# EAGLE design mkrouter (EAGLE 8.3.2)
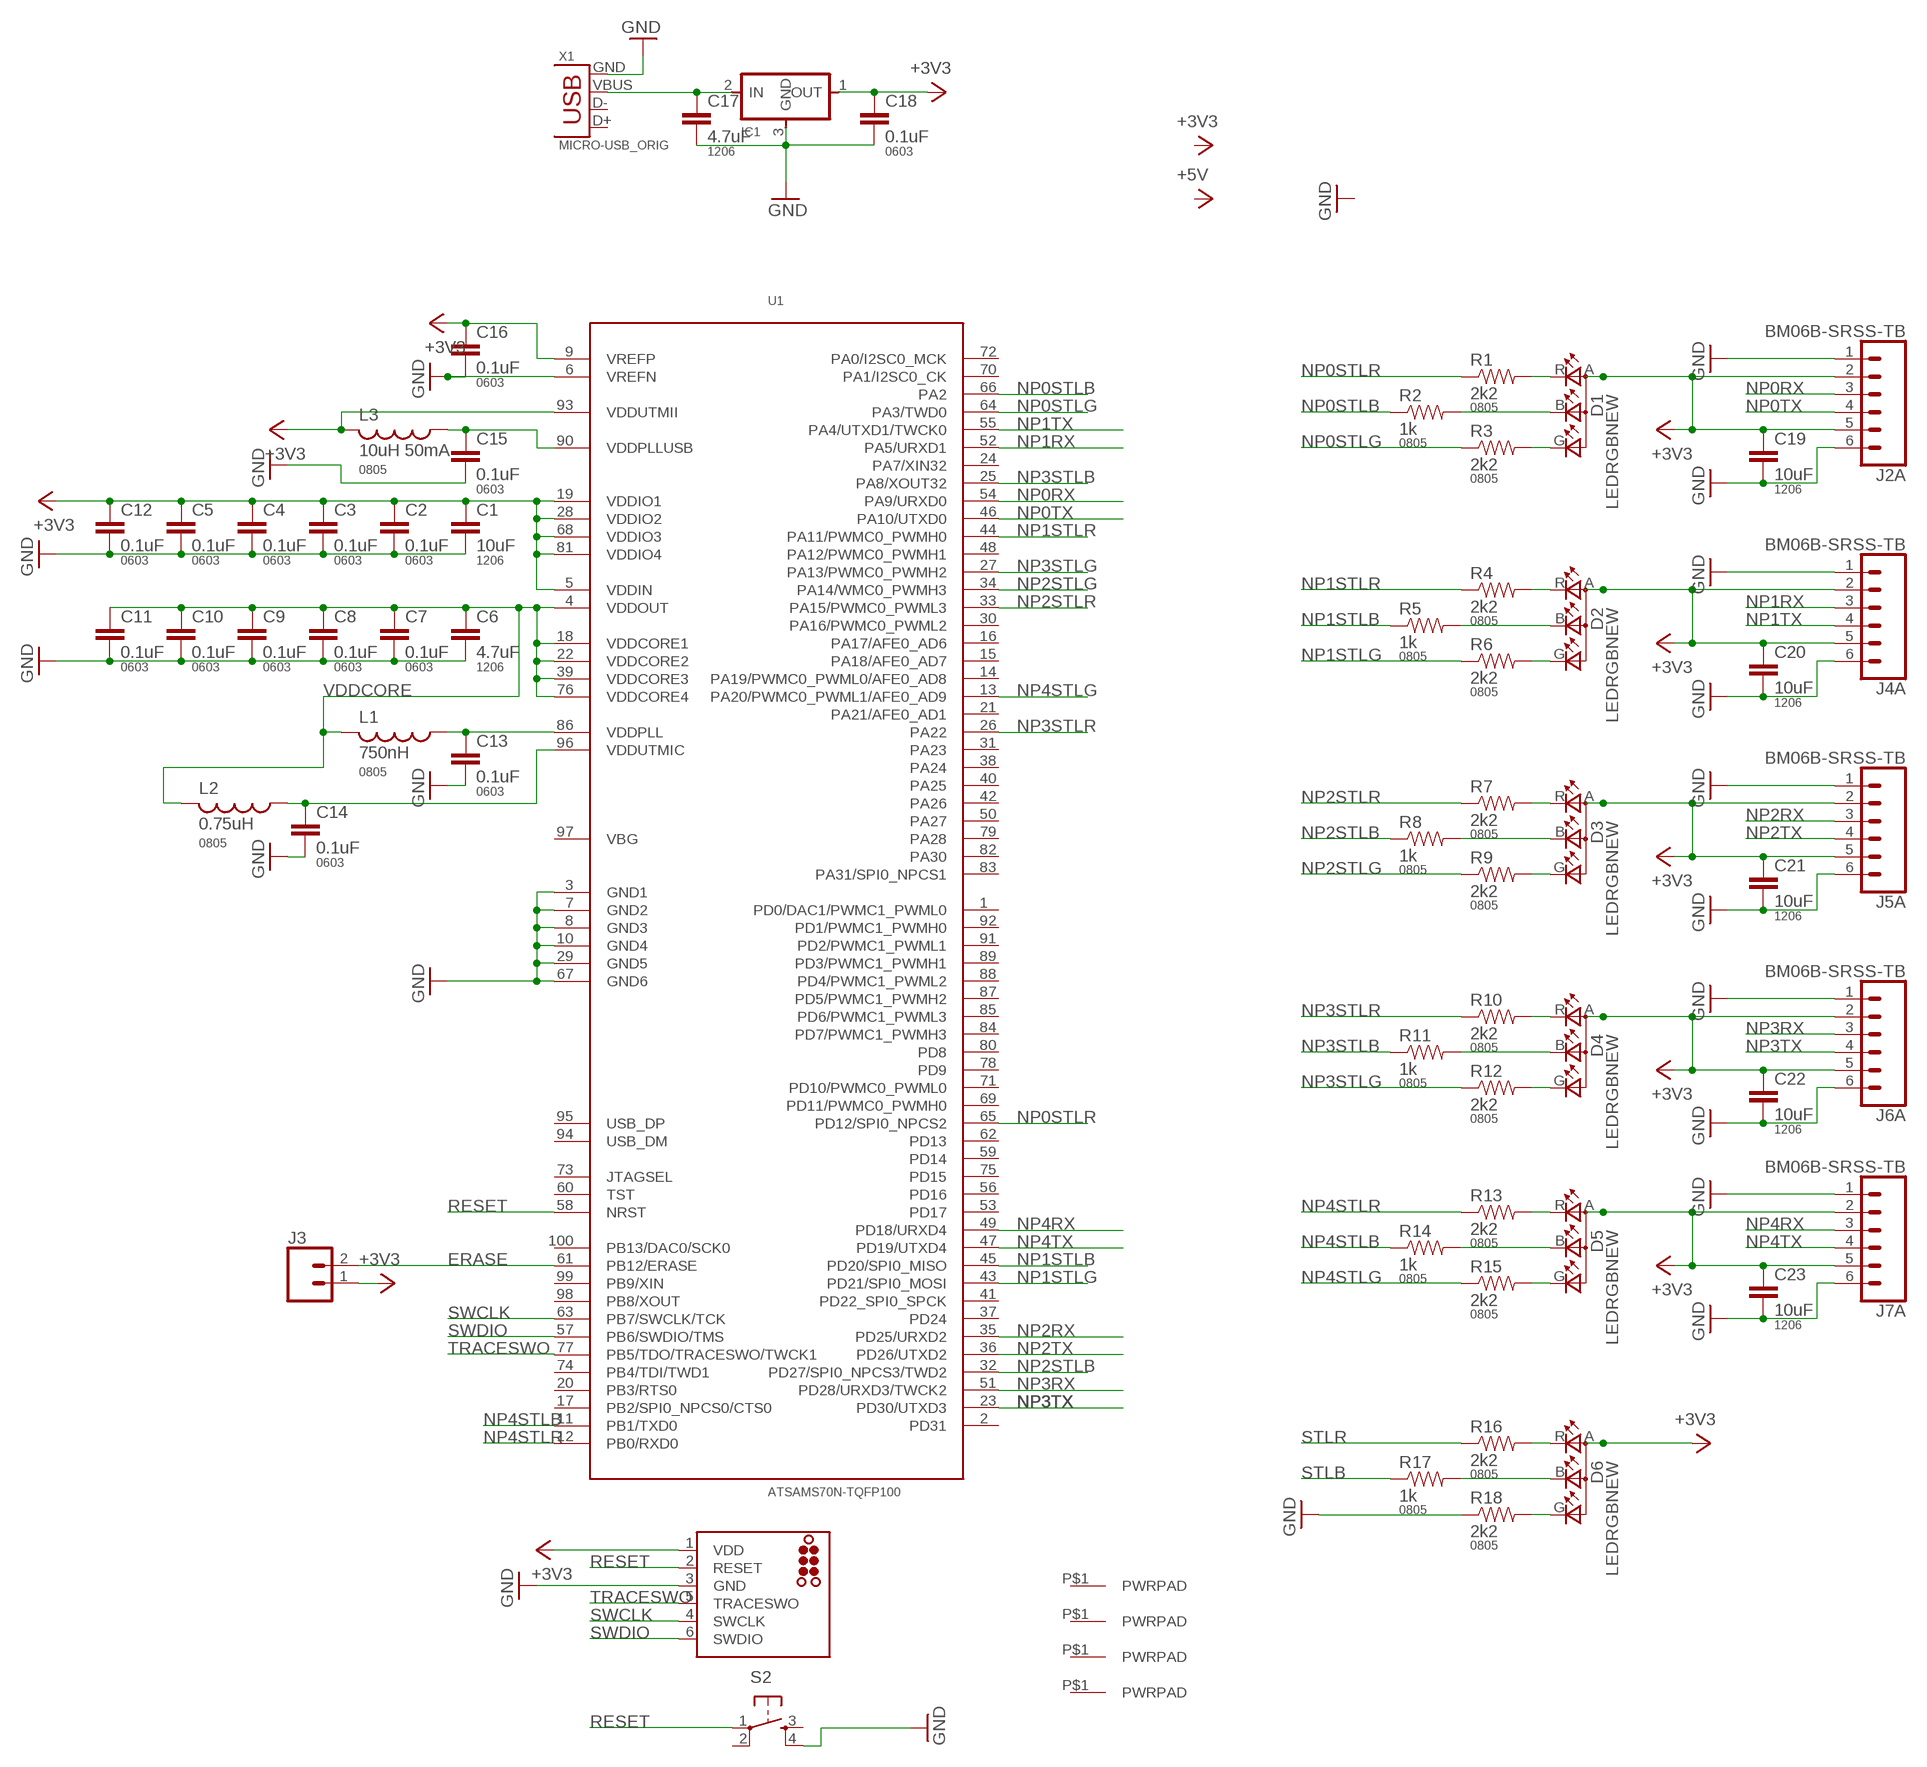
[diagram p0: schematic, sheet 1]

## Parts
C1  10uF  CAP1206  [1206]
C2  0.1uF  CAP0603-CAP  [0603-CAP]
C3  0.1uF  CAP0603-CAP  [0603-CAP]
C4  0.1uF  CAP0603-CAP  [0603-CAP]
C5  0.1uF  CAP0603-CAP  [0603-CAP]
C6  4.7uF  CAP1206  [1206]
C7  0.1uF  CAP0603-CAP  [0603-CAP]
C8  0.1uF  CAP0603-CAP  [0603-CAP]
C9  0.1uF  CAP0603-CAP  [0603-CAP]
C10  0.1uF  CAP0603-CAP  [0603-CAP]
C11  0.1uF  CAP0603-CAP  [0603-CAP]
C12  0.1uF  CAP0603-CAP  [0603-CAP]
C13  0.1uF  CAP0603-CAP  [0603-CAP]
C14  0.1uF  CAP0603-CAP  [0603-CAP]
C15  0.1uF  CAP0603-CAP  [0603-CAP]
C16  0.1uF  CAP0603-CAP  [0603-CAP]
C17  4.7uF  CAP1206  [1206]
C18  0.1uF  CAP0603-CAP  [0603-CAP]
C19  10uF  CAP1206  [1206]
C20  10uF  CAP1206  [1206]
C21  10uF  CAP1206  [1206]
C22  10uF  CAP1206  [1206]
C23  10uF  CAP1206  [1206]
D1  LEDRGBNEW  [P-LCC-4]
D2  LEDRGBNEW  [P-LCC-4]
D3  LEDRGBNEW  [P-LCC-4]
D4  LEDRGBNEW  [P-LCC-4]
D5  LEDRGBNEW  [P-LCC-4]
D6  LEDRGBNEW  [P-LCC-4]
IC1  REGULATORSOT23  [SOT23]
J1  TC2030-SWD-MCP  [TC2030-MCP]
J2  BM06B-SRSS-TB  JST_6_PIN_HORIZONTAL  [JST-6-SMD-HORI-1.0MM]
J3  CONN_021X02_NO_SILK  [1X02_NO_SILK]
J4  BM06B-SRSS-TB  JST_6_PIN_HORIZONTAL  [JST-6-SMD-HORI-1.0MM]
J5  BM06B-SRSS-TB  JST_6_PIN_HORIZONTAL  [JST-6-SMD-HORI-1.0MM]
J6  BM06B-SRSS-TB  JST_6_PIN_HORIZONTAL  [JST-6-SMD-HORI-1.0MM]
J7  BM06B-SRSS-TB  JST_6_PIN_HORIZONTAL  [JST-6-SMD-HORI-1.0MM]
J8  PWRPADM3  [PWRPAD_3-25MM]
J9  PWRPADM3  [PWRPAD_3-25MM]
J10  PWRPADM3  [PWRPAD_3-25MM]
J11  PWRPADM3  [PWRPAD_3-25MM]
L1  750nH  INDUCTOR-0805  [0805]
L2  0.75uH  INDUCTOR-0805  [0805]
L3  10uH 50mA  INDUCTOR-0805  [0805]
R1  2k2  RESISTOR0805-RES  [0805]
R2  1k  RESISTOR0805-RES  [0805]
R3  2k2  RESISTOR0805-RES  [0805]
R4  2k2  RESISTOR0805-RES  [0805]
R5  1k  RESISTOR0805-RES  [0805]
R6  2k2  RESISTOR0805-RES  [0805]
R7  2k2  RESISTOR0805-RES  [0805]
R8  1k  RESISTOR0805-RES  [0805]
R9  2k2  RESISTOR0805-RES  [0805]
R10  2k2  RESISTOR0805-RES  [0805]
R11  1k  RESISTOR0805-RES  [0805]
R12  2k2  RESISTOR0805-RES  [0805]
R13  2k2  RESISTOR0805-RES  [0805]
R14  1k  RESISTOR0805-RES  [0805]
R15  2k2  RESISTOR0805-RES  [0805]
R16  2k2  RESISTOR0805-RES  [0805]
R17  1k  RESISTOR0805-RES  [0805]
R18  2k2  RESISTOR0805-RES  [0805]
S2  6MM_SWITCH6MM_SWITCH  [6MM_SWITCH]
U1  ATSAMS70N-TQFP100  [TQFP100-14X14]
X1  MICRO-USB_ORIG  [DX4R005HJ5]

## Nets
+3V3: C1.1 C2.1 C3.1 C4.1 C5.1 C12.1 C16.1 C18.1 C19.1 C20.1 C21.1 C22.1 C23.1 D1.A(A2) D2.A(A2) D3.A(A2) D4.A(A2) D5.A(A2) D6.A(A2) IC1.1(OUT) J1.1(VDD) J2.2 J2.5 J3.1 J4.2 J4.5 J5.2 J5.5 J6.2 J6.5 J7.2 J7.5 L3.2 U1.5(VDDIN) U1.9(VREFP) U1.19(VDDIO1) U1.28(VDDIO2) U1.68(VDDIO3) U1.81(VDDIO4) U1.93(VDDUTMII)
ERASE: J3.2 U1.61(PB12/ERASE)
GND: C1.2 C2.2 C3.2 C4.2 C5.2 C6.2 C7.2 C8.2 C9.2 C10.2 C11.2 C12.2 C13.2 C14.2 C15.2 C16.2 C17.2 C18.2 C19.2 C20.2 C21.2 C22.2 C23.2 IC1.3(GND) J1.3(GND) J2.1 J2.6 J4.1 J4.6 J5.1 J5.6 J6.1 J6.6 J7.1 J7.6 R18.1 S2.4(S1) U1.3(GND1) U1.6(VREFN) U1.7(GND2) U1.8(GND3) U1.10(GND4) U1.29(GND5) U1.67(GND6) X1.GND
N$1: C13.1 L1.1 U1.86(VDDPLL)
N$2: D1.R(CRED) R1.2
N$3: C14.1 L2.1 U1.96(VDDUTMIC)
N$4: C17.1 IC1.2(IN) X1.VBUS
N$5: C15.1 L3.1 U1.90(VDDPLLUSB)
N$6: D1.B(CBLUE) R2.2
N$7: D1.G(CGREEN) R3.2
N$8: D2.R(CRED) R4.2
N$9: D2.B(CBLUE) R5.2
N$10: D2.G(CGREEN) R6.2
N$11: D3.R(CRED) R7.2
N$12: D3.B(CBLUE) R8.2
N$13: D3.G(CGREEN) R9.2
N$14: D4.R(CRED) R10.2
N$15: D4.B(CBLUE) R11.2
N$16: D4.G(CGREEN) R12.2
N$17: D5.R(CRED) R13.2
N$18: D5.B(CBLUE) R14.2
N$19: D5.G(CGREEN) R15.2
N$20: D6.R(CRED) R16.2
N$21: D6.B(CBLUE) R17.2
N$22: D6.G(CGREEN) R18.2
NP0RX: J2.3 U1.54(PA9/URXD0)
NP0STLB: R2.1 U1.66(PA2)
NP0STLG: R3.1 U1.64(PA3/TWD0)
NP0STLR: R1.1 U1.65(PD12/SPI0_NPCS2)
NP0TX: J2.4 U1.46(PA10/UTXD0)
NP1RX: J4.3 U1.52(PA5/URXD1)
NP1STLB: R5.1 U1.45(PD20/SPI0_MISO)
NP1STLG: R6.1 U1.43(PD21/SPI0_MOSI)
NP1STLR: R4.1 U1.44(PA11/PWMC0_PWMH0)
NP1TX: J4.4 U1.55(PA4/UTXD1/TWCK0)
NP2RX: J5.3 U1.35(PD25/URXD2)
NP2STLB: R8.1 U1.32(PD27/SPI0_NPCS3/TWD2)
NP2STLG: R9.1 U1.34(PA14/WMC0_PWMH3)
NP2STLR: R7.1 U1.33(PA15/PWMC0_PWML3)
NP2TX: J5.4 U1.36(PD26/UTXD2)
NP3RX: J6.3 U1.51(PD28/URXD3/TWCK2)
NP3STLB: R11.1 U1.25(PA8/XOUT32)
NP3STLG: R12.1 U1.27(PA13/PWMC0_PWMH2)
NP3STLR: R10.1 U1.26(PA22)
NP3TX: J6.4 U1.23(PD30/UTXD3)
NP4RX: J7.3 U1.49(PD18/URXD4)
NP4STLB: R14.1 U1.11(PB1/TXD0)
NP4STLG: R15.1 U1.13(PA20/PWMC0_PWML1/AFE0_AD9)
NP4STLR: R13.1 U1.12(PB0/RXD0)
NP4TX: J7.4 U1.47(PD19/UTXD4)
RESET: J1.2(RESET) S2.1(P) U1.58(NRST)
STLB: R17.1
STLR: R16.1
SWCLK: J1.4(SWCLK) U1.63(PB7/SWCLK/TCK)
SWDIO: J1.6(SWDIO) U1.57(PB6/SWDIO/TMS)
TRACESWO: J1.5(TRACESWO) U1.77(PB5/TDO/TRACESWO/TWCK1)
VDDCORE: C6.1 C7.1 C8.1 C9.1 C10.1 C11.1 L1.2 L2.2 U1.4(VDDOUT) U1.18(VDDCORE1) U1.22(VDDCORE2) U1.39(VDDCORE3) U1.76(VDDCORE4)
Unconnected: J2.M1 J2.M2 J4.M1 J4.M2 J5.M1 J5.M2 J6.M1 J6.M2 J7.M1 J7.M2 J8.P$1(PWRPAD) J9.P$1(PWRPAD) J10.P$1(PWRPAD) J11.P$1(PWRPAD) S2.2(P1) S2.3(S) U1.1(PD0/DAC1/PWMC1_PWML0) U1.2(PD31) U1.14(PA19/PWMC0_PWML0/AFE0_AD8) U1.15(PA18/AFE0_AD7) U1.16(PA17/AFE0_AD6) U1.17(PB2/SPI0_NPCS0/CTS0) U1.20(PB3/RTS0) U1.21(PA21/AFE0_AD1) U1.24(PA7/XIN32) U1.30(PA16/PWMC0_PWML2) U1.31(PA23) U1.37(PD24) U1.38(PA24) U1.40(PA25) U1.41(PD22_SPI0_SPCK) U1.42(PA26) U1.48(PA12/PWMC0_PWMH1) U1.50(PA27) U1.53(PD17) U1.56(PD16) U1.59(PD14) U1.60(TST) U1.62(PD13) U1.69(PD11/PWMC0_PWMH0) U1.70(PA1/I2SC0_CK) U1.71(PD10/PWMC0_PWML0) U1.72(PA0/I2SC0_MCK) U1.73(JTAGSEL) U1.74(PB4/TDI/TWD1) U1.75(PD15) U1.78(PD9) U1.79(PA28) U1.80(PD8) U1.82(PA30) U1.83(PA31/SPI0_NPCS1) U1.84(PD7/PWMC1_PWMH3) U1.85(PD6/PWMC1_PWML3) U1.87(PD5/PWMC1_PWMH2) U1.88(PD4/PWMC1_PWML2) U1.89(PD3/PWMC1_PWMH1) U1.91(PD2/PWMC1_PWML1) U1.92(PD1/PWMC1_PWMH0) U1.94(USB_DM) U1.95(USB_DP) U1.97(VBG) U1.98(PB8/XOUT) U1.99(PB9/XIN) U1.100(PB13/DAC0/SCK0) X1.D+ X1.D-

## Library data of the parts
C1 C6 C17 C19-C23 = borkedlabs-passives:CAP: Capacitor; PACKAGE: 1206
C2-C5 C7-C16 C18 = borkedlabs-passives:CAP: Capacitor; PACKAGE: 0603
D1-D6 = fab:LEDRGBNEW
IC1 = fab:REGULATOR
J1 = atsam:TC2030-SWD: TAG-CONNECT ICSP Connector Manufacturer: Tag-Connect Cable for easy In-Circuit Serial Programming. Designed for Microchip ICD2, suitable for many others. Two variants - one "with legs" (for hands-free fit on PCB) and another "without legs" for quick programming. PADDescription 1MCLR/Vpp 2Vdd 3GND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
J2 J4-J7 = SparkFun-Connectors:JST_6_PIN_HORIZONTAL: JST 6 pin horizontal connector JST-SH type. Here is the connector we sell at SparkFun: name (XXX-00000) Datasheet It was used on these SparkFun products: name (XXX-00000) name (XXX-00000); PROD_ID: XXX-00000
J3 = SparkFun-Connectors:CONN_02: Multi connection point. Often used as Generic Header-pin footprint for 0.1 inch spaced/style header connections
J8-J11 = power:PWRPAD
L1-L3 = borkedlabs-passives:INDUCTOR; PACKAGE: 0805
R1-R18 = borkedlabs-passives:RESISTOR: Resistor; PACKAGE: 0805
S2 = fab:6MM_SWITCH: OMRON SWITCH
U1 = atsam:ATSAMS70N-TQFP100
X1 = fab:MICRO-USB: SMD micro USB connector as found in the fablab inventory. Three footprint variants included: original, as described by manufacturer's datasheet for milling with the 1/100" bit for milling with the 1/64" bit Made by Zaerc.

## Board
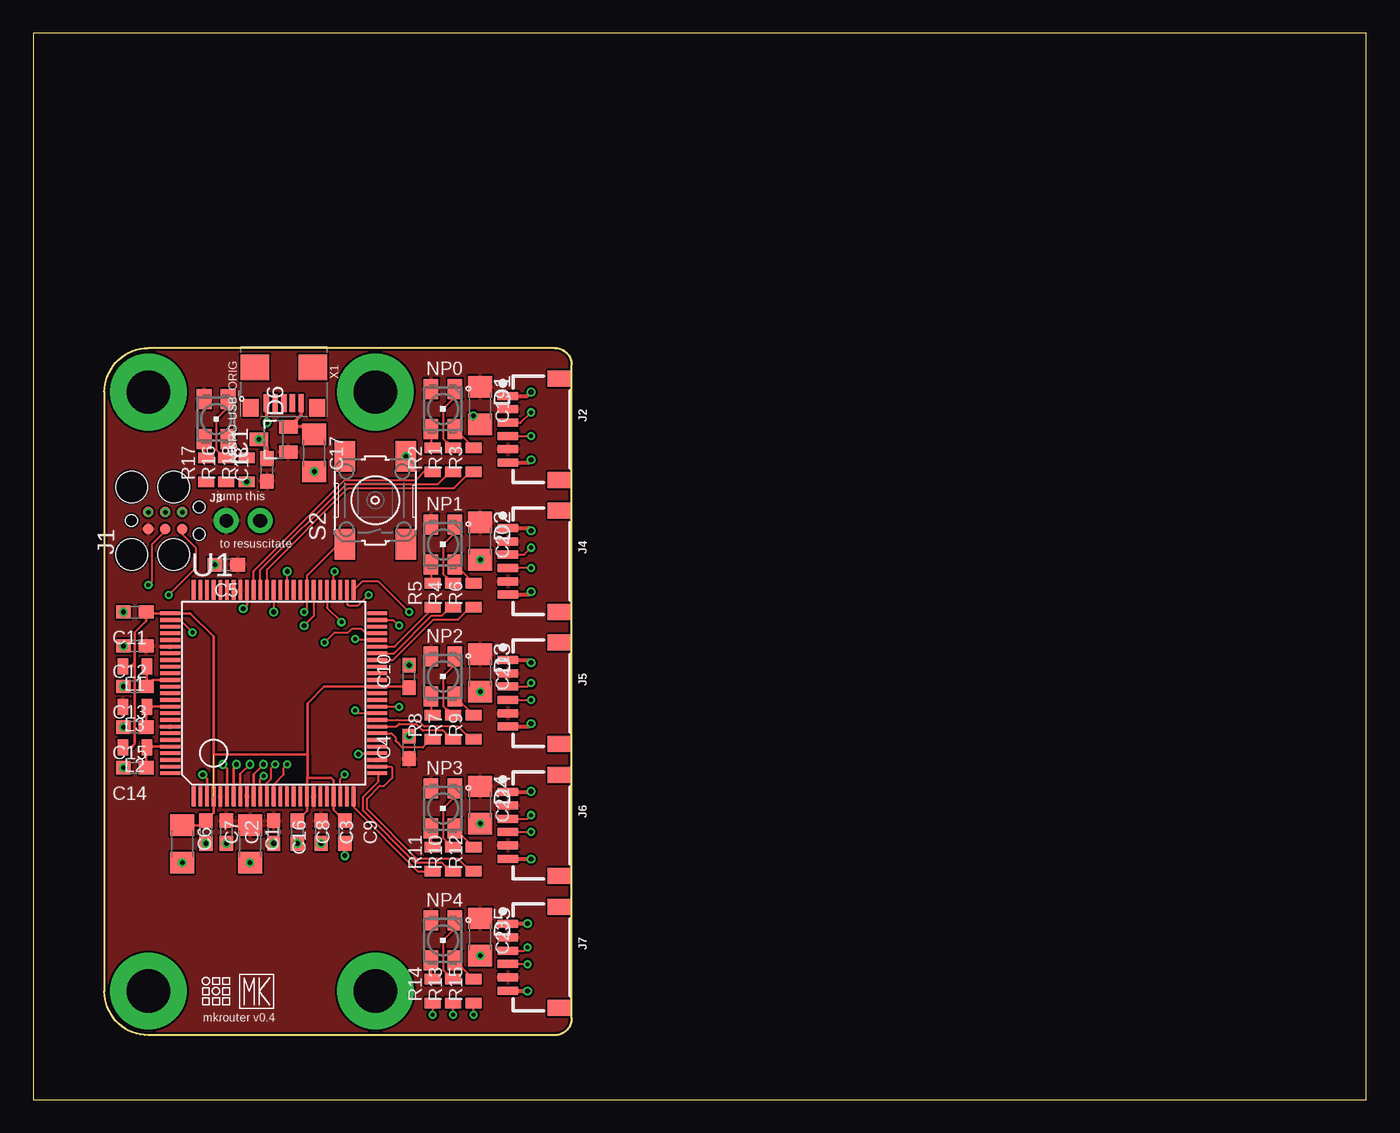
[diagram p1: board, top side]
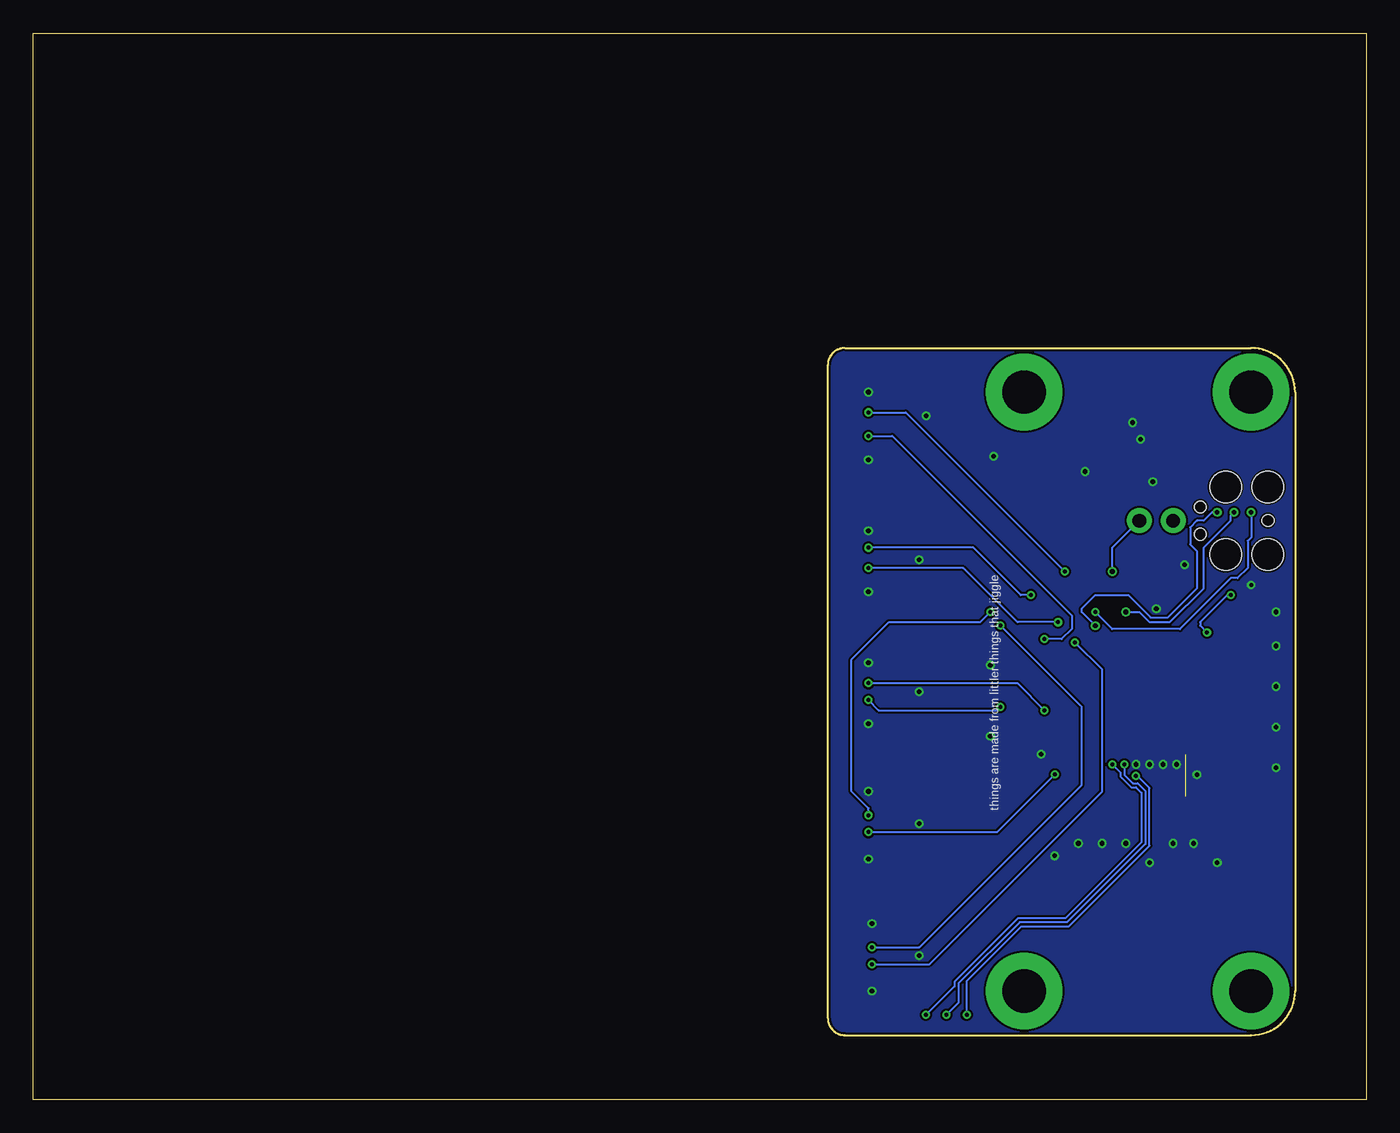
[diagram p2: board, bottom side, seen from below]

Size 100 x 80 mm. Coordinates in mm from the lower left corner, seen from the top.
Outline: 0,0 100,0 100,80 0,80 0,0
Outline: 5.33,53.09 arc-90 8.64,56.39 39.12,56.39 arc-90 40.39,55.12 40.39,6.1 arc-90 39.12,4.83 8.64,4.83 arc-90 5.33,8.13 5.33,53.09
Copper layers (1*16): Top 0.035mm / dielectric 1.5mm / Bottom 0.035mm
Design rules "default *": minimum track width 6mil, minimum drill 0.3mm, track to track 6mil, track to pad 6mil, pad to pad 6mil, via to via 6mil, smd to smd 6mil, copper to edge 6mil, drill to drill 6mil, minimum pad ring 10mil, minimum via ring 6mil, stop-mask expansion 4mil, vias tented up to drill 20mil, thermal gap 6mil

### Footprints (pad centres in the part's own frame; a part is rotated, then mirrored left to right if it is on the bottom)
1206 = smd 1.6 x 1.8: 1 -1.4,0; 2 1.4,0
0603-CAP = smd 1.1 x 1: 1 -0.85,0; 2 0.85,0
P-LCC-4 = smd 1.1 x 1.5: A 0.902,-1.5; B 0.902,1.5; G -0.902,1.5; R -0.902,-1.5
SOT23 = smd 1 x 1.4: 1 -0.95,-1.1; 2 0.95,-1.1; 3 0,1.1
TC2030-MCP = smd 0.787 x 0.787: 1 1.27,-0.635; 2 1.27,0.635; 3 2.54,-0.635; 4 2.54,0.635; 5 3.81,-0.635; 6 3.81,0.635 | hole 0.889: 0,0; 5.08,-1.016; 5.08,1.016 | hole 2.375: 0,2.54; 0,-2.54; 3.175,-2.54; 3.175,2.54
JST-6-SMD-HORI-1.0MM = smd 0.6 x 1.55: 1 -2.5,-4.775; 2 -1.5,-4.775; 3 -0.5,-4.775; 4 0.5,-4.775; 5 1.5,-4.775; 6 2.5,-4.775 | smd 1.2 x 1.8: M1 -3.8,-0.9; M2 3.8,-0.9
1X02_NO_SILK = drill 1.016 pad 1.88: 1 0,0; 2 2.54,0
PWRPAD_3-25MM = drill 3.25 pad 5.75: P$1 0,0
0805 = smd 0.8 x 1.2: 1 -0.9,0; 2 0.9,0
6MM_SWITCH = smd 2.286 x 1.524: 1 -3.302,2.286; 2 3.302,2.286; 3 -3.302,-2.286; 4 3.302,-2.286
TQFP100-14X14 = smd 0.27 x 1.5: 1 -6,-7.75; 2 -5.5,-7.75; 3 -5,-7.75; 4 -4.5,-7.75; 5 -4,-7.75; 6 -3.5,-7.75; 7 -3,-7.75; 8 -2.5,-7.75; 9 -2,-7.75; 10 -1.5,-7.75; 11 -1,-7.75; 12 -0.5,-7.75; 13 0,-7.75; 14 0.5,-7.75; 15 1,-7.75; 16 1.5,-7.75; 17 2,-7.75; 18 2.5,-7.75; 19 3,-7.75; 20 3.5,-7.75; 21 4,-7.75; 22 4.5,-7.75; 23 5,-7.75; 24 5.5,-7.75; 25 6,-7.75; 51 6,7.75; 52 5.5,7.75; 53 5,7.75; 54 4.5,7.75; 55 4,7.75; 56 3.5,7.75; 57 3,7.75; 58 2.5,7.75; 59 2,7.75; 60 1.5,7.75; 61 1,7.75; 62 0.5,7.75; 63 0,7.75; 64 -0.5,7.75; 65 -1,7.75; 66 -1.5,7.75; 67 -2,7.75; 68 -2.5,7.75; 69 -3,7.75; 70 -3.5,7.75; 71 -4,7.75; 72 -4.5,7.75; 73 -5,7.75; 74 -5.5,7.75; 75 -6,7.75 | smd 1.5 x 0.27: 26 7.75,-6; 27 7.75,-5.5; 28 7.75,-5; 29 7.75,-4.5; 30 7.75,-4; 31 7.75,-3.5; 32 7.75,-3; 33 7.75,-2.5; 34 7.75,-2; 35 7.75,-1.5; 36 7.75,-1; 37 7.75,-0.5; 38 7.75,0; 39 7.75,0.5; 40 7.75,1; 41 7.75,1.5; 42 7.75,2; 43 7.75,2.5; 44 7.75,3; 45 7.75,3.5; 46 7.75,4; 47 7.75,4.5; 48 7.75,5; 49 7.75,5.5; 50 7.75,6; 76 -7.75,6; 77 -7.75,5.5; 78 -7.75,5; 79 -7.75,4.5; 80 -7.75,4; 81 -7.75,3.5; 82 -7.75,3; 83 -7.75,2.5; 84 -7.75,2; 85 -7.75,1.5; 86 -7.75,1; 87 -7.75,0.5; 88 -7.75,0; 89 -7.75,-0.5; 90 -7.75,-1; 91 -7.75,-1.5; 92 -7.75,-2; 93 -7.75,-2.5; 94 -7.75,-3; 95 -7.75,-3.5; 96 -7.75,-4; 97 -7.75,-4.5; 98 -7.75,-5; 99 -7.75,-5.5; 100 -7.75,-6
DX4R005HJ5 = smd 0.4 x 1.35: D+ 0,1.6; D- -0.65,1.6; GND 1.3,1.6; ID 0.65,1.6; VBUS -1.3,1.6 | smd 1.2 x 1.3: GND@1 -2.5,1.95; GND@2 2.5,1.95 | smd 2.15 x 1.9: GND@3 -2.175,-1.1; GND@4 2.175,-1.1

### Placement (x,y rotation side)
C1  16.26,19.18 270 top
C2  14.48,20.07 270 top
C3  21.59,20.07 270 top
C4  28.19,26.42 90 top
C5  14.48,40.13 180 top
C6  11.18,19.18 270 top
C7  12.95,20.07 270 top
C8  19.81,20.07 270 top
C9  23.37,20.07 270 top
C10  28.19,31.75 90 top
C11  7.62,36.58 180 top
C12  7.62,34.04 180 top
C13  7.62,30.99 180 top
C14  7.62,24.89 180 top
C15  7.62,27.94 180 top
C16  18.03,20.07 270 top
C17  21.08,48.51 270 top
C18  17.53,47.24 90 top
C19  33.53,52.07 270 top
C20  33.53,41.91 270 top
C21  33.53,32 270 top
C22  33.53,22.1 270 top
C23  33.53,12.19 270 top
D1  30.73,51.82 180 top
D2  30.73,41.66 180 top
D3  30.73,31.75 180 top
D4  30.73,21.84 180 top
D5  30.73,11.94 180 top
D6  13.72,51.05 180 top
IC1  18.03,49.53 90 top
J1  7.37,43.43 0 top
J2  40.39,50.29 270 top
J3  14.48,43.43 0 top
J4  40.39,40.39 270 top
J5  40.39,30.48 270 top
J6  40.39,20.57 270 top
J7  40.39,10.67 270 top
J8  8.64,8.13 0 top
J9  25.65,8.13 0 top
J10  25.65,53.09 0 top
J11  8.64,53.09 0 top
L1  7.62,32.51 180 top
L2  7.62,26.42 180 top
L3  7.62,29.46 180 top
R1  31.5,48.01 90 top
R2  29.97,48.01 90 top
R3  33.02,48.01 90 top
R4  31.5,37.85 90 top
R5  29.97,37.85 90 top
R6  33.02,37.85 90 top
R7  31.5,27.94 90 top
R8  29.97,27.94 90 top
R9  33.02,27.94 90 top
R10  31.5,18.03 90 top
R11  29.97,18.03 90 top
R12  33.02,18.03 90 top
R13  31.5,8.13 90 top
R14  29.97,8.13 90 top
R15  33.02,8.13 90 top
R16  14.48,47.24 90 top
R17  12.95,47.24 90 top
R18  16,47.24 90 top
S2  25.65,44.96 90 top
U1  18.03,30.48 0 top
U$1  [CBA-SILK-LOGO]  13.72,8.13 0 top
U$2  [MK-LOGO-SILK]  16.76,8.13 0 top
X1  18.8,53.85 180 top

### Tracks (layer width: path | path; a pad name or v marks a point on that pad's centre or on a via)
+3V3
  pour Top (rank 2): 5.33,56.39 5.33,4.83 40.39,4.83 40.39,56.39
ERASE  (via drill 0.35)
  Top 0.152: U1.61 19.03,39.61 v19.05,39.62
  Bottom 0.152: v19.05,39.62 19.05,41.4 J3.2
GND  (via drill 0.3, 0.35)
  Top 0.152: C9.2 v23.37,18.29 | J1.3 9.91,42.67 8.89,41.66 8.89,38.86 v8.64,38.61
  Top 0.203: U1.3 13.03,24.05 v12.7,24.38 | U1.6 14.53,24.84 v14.22,25.15 | U1.7 15.03,24.94 v15.24,25.15 | U1.8 15.53,24.42 v16.26,25.15 | U1.10 16.53,24.41 v17.27,25.15 | U1.67 16.03,37.12 v15.75,36.83 | U1.29 24.46,25.98 v24.38,25.91
  Top 0.254: C18.2 17.53,48.94 IC1.3 | X1.GND 17.5,50.83 v17.53,50.8
  Top 0.305: J5.1 37.12,32.98 v37.34,32.77 | J5.6 37.12,27.98 v37.34,28.19 | J4.6 37.12,37.89 v37.34,38.1 | J4.1 37.12,42.89 v37.34,42.67 | J2.6 37.12,47.79 v37.34,48.01 | J2.1 37.04,52.79 v37.34,53.09 | J6.1 37.3,23.07 v37.34,23.11 | J6.6 37.3,18.07 v37.34,18.03 | J7.1 37.04,13.17 v37.08,13.21 | J7.6 37.04,8.17 v37.08,8.13 | C19.2 33.53,50.8 v33.02,51.31
  other vias: 6.77,36.58 6.77,34.04 6.77,30.99 6.77,27.94 6.77,24.89 16.93,49.53 21.08,47.11 16,46.34 13.63,40.13 11.18,17.78 12.95,19.22 14.48,19.22 16.26,17.78 18.03,19.22 19.81,19.22 21.59,19.22 28.19,27.27 28.19,32.6 27.94,48.26 33.53,10.79 33.53,20.7 33.53,30.6 33.53,40.51
  pour Bottom: 5.33,56.39 40.39,56.39 40.39,4.83 5.33,4.83
N$1
  Top 0.203: 8.52,31.04 L1.1 | 8.52,31.04 C13.1 | U1.86 8.96,31.48 8.52,31.04
N$2
  Top 0.152: D1.R 31.64,52.72 30.73,51.82 30.73,49.59 30.99,49.34 31.07,49.34 R1.2
N$3
  Top 0.203: U1.96 8.58,26.48 L2.1 8.47,26.37 C14.1
N$4
  Top 0.254: X1.VBUS 20.1,51.34 19.24,50.48 IC1.2 20.52,50.48 C17.1
N$5
  Top 0.203: U1.90 8.54,29.48 L3.1 8.47,29.41 C15.1
N$6
  Top 0.152: D1.B 29.83,49.05 R2.2
N$7
  Top 0.152: D1.G 31.64,50.29 R3.2
N$8
  Top 0.152: D2.R 31.64,42.56 30.73,41.66 30.73,39.43 30.99,39.18 31.07,39.18 R4.2
N$9
  Top 0.152: D2.B 29.83,38.89 R5.2
N$10
  Top 0.152: D2.G 31.64,40.13 R6.2
N$11
  Top 0.152: D3.R 31.64,32.65 30.73,31.75 30.73,29.53 30.99,29.27 31.07,29.27 R7.2
N$12
  Top 0.152: D3.B 29.83,28.98 R8.2
N$13
  Top 0.152: D3.G 31.64,30.22 R9.2
N$14
  Top 0.152: D4.R 31.64,22.75 30.73,21.84 30.73,19.62 30.99,19.36 31.07,19.36 R10.2
N$15
  Top 0.152: D4.B 29.83,19.07 R11.2
N$16
  Top 0.152: D4.G 31.64,20.32 R12.2
N$17
  Top 0.152: D5.R 31.64,12.84 30.73,11.94 30.73,9.72 30.99,9.46 31.07,9.46 R13.2
N$18
  Top 0.152: D5.B 29.83,9.17 R14.2
N$19
  Top 0.152: D5.G 31.64,10.41 R15.2
N$20
  Top 0.152: D6.R 14.62,51.96 13.72,51.05 13.72,48.77 13.97,48.51 14.11,48.51 R16.2
N$21
  Top 0.152: D6.B 12.81,48.28 R17.2
N$22
  Top 0.152: R18.2 16,48.17 D6.G
NP0RX  (via drill 0.3)
  Top 0.152: J2.3 36.57,50.79 v37.34,51.56 | U1.54 22.53,39.55 v22.61,39.62
  Bottom 0.152: v37.34,51.56 34.54,51.56 v22.61,39.62
NP0STLB
  Top 0.152: R2.1 29.33,47.11 28.7,46.48 23.37,46.48 16.53,39.65 U1.66
NP0STLG
  Top 0.152: R3.1 32.82,47.11 31.59,45.87 23.62,45.87 17.53,39.79 U1.64
NP0STLR
  Top 0.152: R1.1 31.3,47.11 30.37,46.18 23.49,46.18 17.03,39.72 U1.65
NP0TX  (via drill 0.3)
  Top 0.152: J2.4 37.33,49.79 v37.34,49.78 | U1.46 24.19,34.48 v24.13,34.54
  Bottom 0.152: v37.34,49.78 35.56,49.78 22.1,36.32 22.1,35.31 22.86,34.54 v24.13,34.54
NP1RX  (via drill 0.3)
  Top 0.152: U1.52 23.53,37.17 23.62,37.08 24.38,37.08 v25.15,37.85 | J4.3 36.82,40.89 v37.34,41.4
  Bottom 0.152: v25.15,37.85 25.91,37.85 29.46,41.4 v37.34,41.4
NP1STLB
  Top 0.152: R5.1 29.97,36.83 27.12,33.98 U1.45
NP1STLG
  Top 0.152: R6.1 32.82,36.95 31.89,36.01 30.02,36.01 26.98,32.98 U1.43
NP1STLR
  Top 0.152: R4.1 31.3,36.95 30.67,36.32 29.89,36.32 27.05,33.48 U1.44
NP1TX  (via drill 0.3)
  Top 0.152: U1.55 22.03,36.89 v23.11,35.81 | v37.34,39.88 35.62,39.88 J4.4
  Bottom 0.152: v23.11,35.81 26.16,35.81 30.23,39.88 v37.34,39.88
NP2RX  (via drill 0.3)
  Top 0.152: J5.3 37.08,30.98 v37.34,31.24 | U1.35 24.36,28.98 v24.13,29.21
  Bottom 0.152: v37.34,31.24 26.16,31.24 v24.13,29.21
NP2STLB
  Top 0.152: R8.1 29.83,27.04 29.21,26.42 27.67,26.42 27.46,26.62 27.46,26.64 27.18,26.92 27.18,27.18 26.88,27.48 U1.32
NP2STLG
  Top 0.152: R9.1 32.82,27.04 31.87,27.99 29.34,27.99 28.83,28.5 27.31,28.5 27.29,28.48 U1.34
NP2STLR
  Top 0.152: R7.1 31.38,27.04 30.73,27.69 29.21,27.69 28.7,28.19 27.43,28.19 27.22,27.98 U1.33
NP2TX  (via drill 0.3)
  Top 0.152: J5.4 v37.33,29.98 v37.34,29.97 | v27.43,29.46 25.8,29.46 U1.36
  Bottom 0.152: v37.34,29.97 36.58,29.21 27.69,29.21 v27.43,29.46
NP3RX  (via drill 0.3)
  Top 0.152: J6.3 37.08,21.07 v37.34,21.34 | v28.19,36.58 25.91,38.86 24.67,38.86 U1.51
  Bottom 0.152: v37.34,21.34 37.34,21.84 38.61,23.11 38.61,33.02 35.81,35.81 28.96,35.81 v28.19,36.58
NP3STLB
  Top 0.152: R11.1 28.84,17.13 24.03,21.94 U1.25
NP3STLG
  Top 0.152: R12.1 32.82,17.13 31.89,18.07 28.77,18.07 25.03,21.8 25.03,22.57 26,23.53 26.33,23.53 26.92,24.13 26.92,24.89 26.84,24.98 U1.27
NP3STLR
  Top 0.152: R10.1 31.3,17.13 30.67,17.76 28.64,17.76 24.73,21.68 24.73,22.7 25.91,23.88 25.91,24.36 U1.26
NP3TX  (via drill 0.3)
  Top 0.152: J6.4 v37.33,20.07 v37.34,20.07 | U1.23 23.03,24.05 v23.37,24.38
  Bottom 0.152: v37.34,20.07 27.69,20.07 v23.37,24.38
NP4RX  (via drill 0.3)
  Top 0.152: J7.3 36.82,11.17 v37.08,11.43 | U1.49 27.01,35.98 v27.43,35.56
  Bottom 0.152: v37.08,11.43 33.53,11.43 21.34,23.62 21.34,29.46 v27.43,35.56
NP4STLB  (via drill 0.3)
  Top 0.152: R14.1 v29.97,6.35 | U1.11 17.03,24.05 v17.27,24.29
  Bottom 0.152: v29.97,6.35 29.97,8.89 25.87,12.99 22.31,12.99 16.26,19.05 16.26,23.37 17.02,24.13 17.11,24.13 v17.27,24.29
NP4STLG  (via drill 0.3)
  Top 0.152: U1.13 18.03,23.62 18.8,24.38 18.8,24.89 v19.05,25.15 | v33.02,6.35 R15.1
  Bottom 0.152: v19.05,25.15 18.44,24.53 18.44,24.23 17.63,23.43 17.27,23.43 16.87,23.02 16.87,19.3 22.57,13.6 26.12,13.6 30.88,8.84 30.88,8.49 v33.02,6.35
NP4STLR  (via drill 0.3)
  Top 0.152: v31.5,6.35 R13.1 | U1.12 17.53,23.76 17.83,24.06 17.83,24.84 v18.13,25.15
  Bottom 0.152: v31.5,6.35 30.58,7.27 30.58,8.71 26,13.3 22.44,13.3 16.56,19.18 16.56,23.14 17.15,23.73 17.5,23.73 18.13,24.36 v18.13,25.15
NP4TX  (via drill 0.3)
  Top 0.152: J7.4 v37.08,10.17 v37.08,10.16 | v21.84,34.29 22.61,35.05 23.62,35.05 23.88,35.31 24.64,35.31 24.96,34.98 U1.47
  Bottom 0.152: v37.08,10.16 32.77,10.16 19.81,23.11 19.81,32.26 v21.84,34.29
RESET  (via drill 0.3, 0.35)
  Top 0.152: v20.32,36.58 20.53,36.79 U1.58 20.53,39.33 22.86,41.66 S2.1
  Bottom 0.152: J1.2 8.64,42.16 8.89,41.91 8.89,39.88 9.65,39.12 10.16,39.12 13.97,35.31 19.05,35.31 v20.32,36.58
  other vias: 8.64,44.07
SWCLK  (via drill 0.35)
  Top 0.152: U1.63 v18.03,36.58
  Bottom 0.152: v18.03,36.58 17.02,36.58 16.26,35.81 14.73,35.81 12.19,38.35 12.19,41.4 10.16,43.43 10.16,43.81 J1.4
  other vias: 9.91,44.07
SWDIO  (via drill 0.35)
  Top 0.152: U1.57 21.03,36.27 v20.32,35.56
  Bottom 0.152: v20.32,35.56 21.34,36.58 21.34,36.83 20.32,37.85 17.86,37.85 16.17,36.16 14.9,36.16 12.7,38.35 12.7,41.15 13.21,41.66 13.21,42.93 12.7,43.43 12.19,43.43 11.56,44.07 J1.6
  other vias: 11.18,44.07
TRACESWO  (via drill 0.3)
  Top 0.152: J1.5 11.18,42.42 12.19,41.4 12.19,39.88 v10.16,37.85 | U1.77 11.01,35.98 v11.94,35.05
  Bottom 0.152: v10.16,37.85 10.41,37.85 12.45,35.81 12.45,35.56 v11.94,35.05
VDDCORE  (1 unrouted)
  Top 0.203: 7.62,32.77 7.62,35.05 8.47,35.9 C11.1 8.57,36.48 U1.76 11.78,36.48 13.53,34.73 U1.4 13.53,21.5 C7.1 12.62,20.58 C6.1 | 7.62,32.77 7.37,32.51 L1.2 | 7.62,32.77 7.62,26.67 7.37,26.42 L2.2 | C8.1 20.53,21.64 U1.18 20.53,24.13 | C9.1 22.53,21.75 U1.22 22.53,23.95 22.35,24.13 20.53,24.13 | 20.53,24.13 20.53,24.17 | 20.57,25.91 20.57,29.72 21.84,30.98 U1.39 28.11,30.98 C10.1 | 20.57,25.91 20.57,24.17 20.53,24.13 | 13.53,25.91 20.57,25.91

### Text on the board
tPlace: NP0 | jump this | NP1 | to resuscitate | NP2 | NP3 | NP4 | mkrouter v0.4
bPlace: things are made from littler things that jiggle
